VAR_GLOBAL CONSTANT
	
	cOversamples 	: UDINT 	:= 10;		// number of oversamples
	cFFTLength		: UDINT		:= 2048;	// length of FFT 
	cBufferLength	: UDINT		:= cFFTLength;	    // buffer size - needs to be equal to cFFTLength	
	cFFTResult 		: UDINT 	:= cFFTLength;	// result of spectrum (full length; not N/2+1) -> see Scope
		
END_VAR
